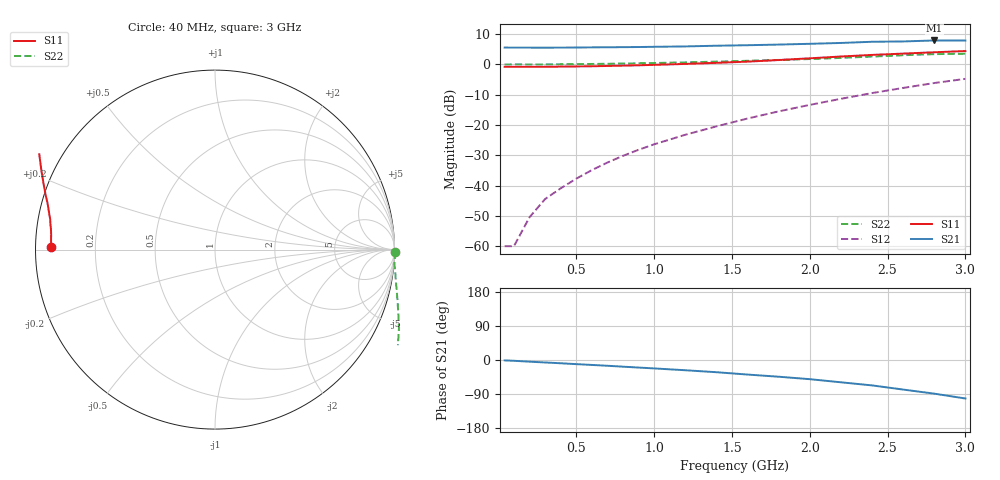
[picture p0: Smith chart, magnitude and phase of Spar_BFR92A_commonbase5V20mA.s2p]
! Filename:  BFR92ACE.S2P  Version:  2.0
! NXP part #: BFR92A  Date: Jul 1990
! Bias condition: Vce=5V, Ic=20mA
! COMMON BASE
#  MHz  S  MA  R  50
! Freq  S11  S21  S12  S22
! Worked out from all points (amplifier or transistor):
!   21 points, 40 MHz to 3 GHz, reference 50 ohm
!   highest |S21| = 7.9 dB at 2.8 GHz (marker M1)
!   |S21| within 3 dB of that: start of sweep to end of sweep
!   unconditionally stable (mu >= 1): nowhere
!   at 300 MHz: K = -0.63, MSG = 25.0 dB, |S12| = -44.4 dB
!   at 1 GHz: K = -0.95, MSG = 16.1 dB, |S12| = -26.4 dB
!   at 3 GHz: K = -0.89, MSG = 6.3 dB, |S12| = -4.7 dB
40  0.915 179.2  1.901 -1.0  0.001 60.5  1.002 -0.7
100  0.914 178.1  1.899 -2.1  0.001 83.5  1.004 -1.4
200  0.915 176.3  1.897 -4.4  0.003 112.4  1.003 -3.0
300  0.917 174.6  1.895 -6.5  0.006 126.5  1.003 -4.6
400  0.921 172.9  1.898 -8.6  0.009 136.6  1.008 -6.1
500  0.928 171.2  1.905 -10.9  0.013 138.5  1.014 -7.7
600  0.934 169.5  1.916 -13.0  0.018 142.8  1.02 -9.2
700  0.945 167.8  1.924 -15.2  0.024 145.6  1.027 -10.8
800  0.957 166.0  1.931 -17.6  0.031 147.0  1.036 -12.3
900  0.969 164.4  1.941 -19.9  0.039 148.2  1.046 -14.1
1000  0.986 162.7  1.958 -22.2  0.048 148.7  1.057 -15.8
1200  1.021 159.2  1.986 -27.0  0.069 149.3  1.083 -19.4
1400  1.063 155.5  2.04 -32.2  0.095 148.0  1.115 -23.2
1600  1.114 151.5  2.079 -38.4  0.128 146.9  1.15 -27.6
1800  1.183 147.4  2.131 -44.1  0.168 144.2  1.189 -32.4
2000  1.264 143.1  2.194 -50.6  0.215 141.2  1.229 -38.2
2200  1.353 138.5  2.266 -58.8  0.271 137.4  1.283 -45.1
2400  1.438 133.2  2.371 -67.0  0.337 132.6  1.35 -52.7
2600  1.512 126.3  2.399 -78.0  0.41 127.3  1.421 -61.0
2800  1.59 117.7  2.492 -88.8  0.494 120.2  1.481 -69.6
3000  1.667 108.4  2.485 -101.6  0.579 113.0  1.506 -79.3
